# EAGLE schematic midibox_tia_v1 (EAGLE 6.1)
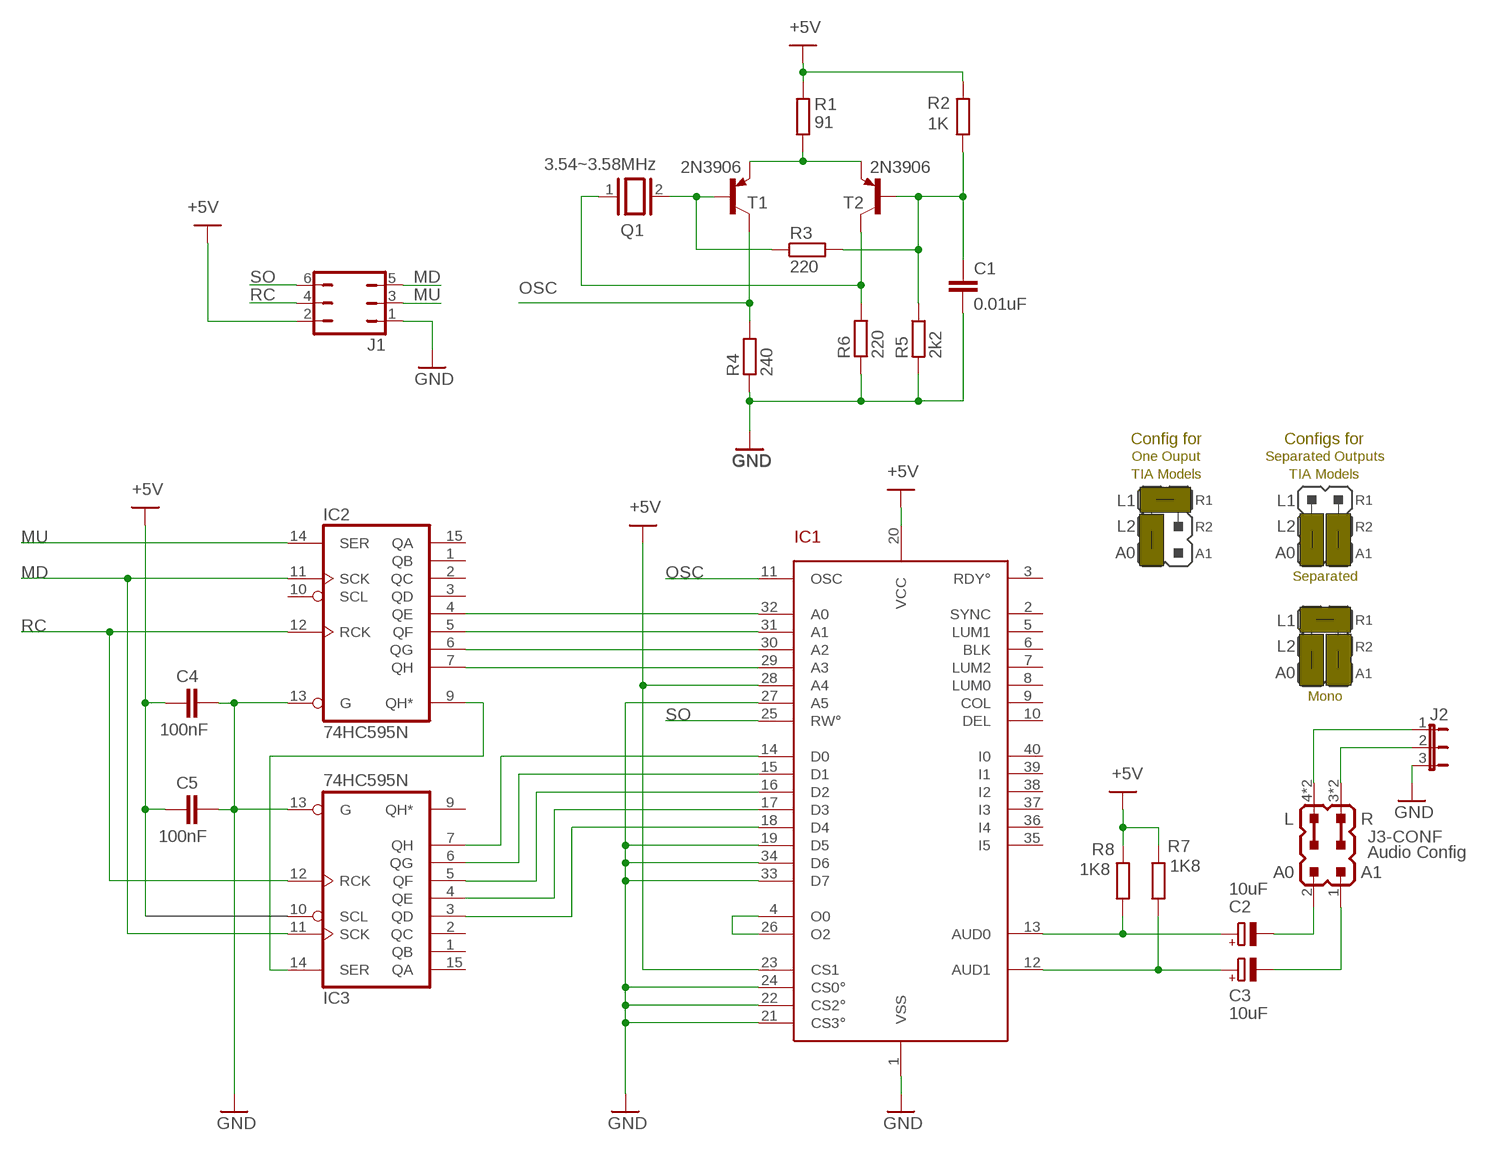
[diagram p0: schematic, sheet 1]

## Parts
C1  0.01uF  MYTYNYC  [MYC]
C2  10uF  CPOL-EUE2.5-5  [E2,5-5]
C3  10uF  CPOL-EUE2.5-5  [E2,5-5]
C4  100nF  MYTYNYC  [MYC]
C5  100nF  MYTYNYC  [MYC]
IC1  TIA_C011903  [ATARI_DIL40]
IC2  74HC595N  [DIL16]
IC3  74HC595N  [DIL16]
J1  JP3Q  [JP3Q]
J2  JP2E  [JP2]
J3  Audio Config  JP-TIA_AUDOUT_CONF  [JP3Q]
Q1  3.54~3.58MHz  XTAL/S  [QS]
R1  91  R-EU_0207/2V  [0207/2V]
R2  1K  R-EU_0207/2V  [0207/2V]
R3  220  R-EU_0207/2V  [0207/2V]
R4  240  R-EU_0207/2V  [0207/2V]
R5  2k2  R-EU_0207/2V  [0207/2V]
R6  220  R-EU_0207/2V  [0207/2V]
R7  1K8  R-EU_0207/5V  [0207/5V]
R8  1K8  R-EU_0207/2V  [0207/2V]
T1  2N3906  [TO92]
T2  2N3906  [TO92]

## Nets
+5V: C4.1 C5.1 IC1.20(VCC) IC1.23(CS1) IC1.28(A4) J1.2 R1.1 R2.1 R7.1 R8.1
GND: C4.2 C5.2 IC1.1(VSS) IC1.19(D5) IC1.21(CS3°) IC1.22(CS2°) IC1.24(CS0°) IC1.27(A5) IC1.33(D7) IC1.34(D6) IC2.13(G) IC3.13(G) J1.1 J2.3
MD: IC2.11(SCK) IC3.11(SCK) J1.5
MU: IC2.14(SER) J1.3
N$1: R1.2 T1.3(E) T2.3(E)
N$2: Q1.2 R3.1 T1.2(B)
N$3: IC1.32(A0) IC2.4(QE)
N$4: C2.+ IC1.13(AUD0) R8.2
N$5: Q1.1 R6.2 T2.1(C)
N$6: IC1.31(A1) IC2.5(QF)
N$7: C1.1 R2.2 R3.2 R5.1 T2.2(B)
N$8: IC1.30(A2) IC2.6(QG)
N$9: IC1.29(A3) IC2.7(QH)
N$10: C3.+ IC1.12(AUD1) R7.2
N$11: IC1.14(D0) IC3.7(QH)
N$12: IC1.18(D4) IC3.3(QD)
N$13: IC1.15(D1) IC3.6(QG)
N$14: IC1.16(D2) IC3.5(QF)
N$15: IC1.17(D3) IC3.4(QE)
N$16: C2.- J3.2(-CONF:A0)
N$17: C3.- J3.1(-CONF:A1)
N$18: IC2.9(QH*) IC3.14(SER)
N$19: J2.1 J3.4(-CONF:L1) J3.6(-CONF:L1)
N$20: J2.2 J3.3(-CONF:R1) J3.5(-CONF:R1)
N$28: IC1.4(O0) IC1.26(O2)
OSC: IC1.11(OSC) R4.1 T1.1(C)
R6: C1.2 R4.2 R5.2 R6.1 ; supply symbol labelled GND
RC: IC2.12(RCK) IC3.12(RCK) J1.4
SO: IC1.25(RW°) J1.6
Unconnected: IC1.2(SYNC) IC1.3(RDY°) IC1.5(LUM1) IC1.6(BLK) IC1.7(LUM2) IC1.8(LUM0) IC1.9(COL) IC1.10(DEL) IC1.35(I5) IC1.36(I4) IC1.37(I3) IC1.38(I2) IC1.39(I1) IC1.40(I0) IC2.1(QB) IC2.2(QC) IC2.3(QD) IC2.10(SCL) IC2.15(QA) IC3.1(QB) IC3.2(QC) IC3.9(QH*) IC3.10(SCL) IC3.15(QA)

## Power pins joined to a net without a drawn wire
GND: IC2.8(GND) IC3.8(GND)
VCC: IC2.16(VCC) IC3.16(VCC)

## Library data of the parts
C1 C4 C5 = rcl:MYTYNYC
C2 C3 = rcl:CPOL-EU: POLARIZED CAPACITOR, European symbol
IC1 = atari_chipsets:TIA_C011903
IC2 IC3 = 74xx-eu:74*595: 8-bit SHIFT REGISTER, output latch
J1 = jumper:JP3Q: JUMPER
J2 = jumper:JP2E: JUMPER
J3 = atari_chipsets:JP-TIA_AUDOUT_CONF: Configuration JUMPER for TIA Audio Outputs
Q1 = special:XTAL/S: CRYSTAL
R1-R8 = resistor:R-EU_: RESISTOR, European symbol
T1 T2 = transistor-pnp:2N3906: PNP Transistor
